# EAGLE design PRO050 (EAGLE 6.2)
CHECKED: PJC; DATE: 9/8/09; DRAWN: PJC; DRGNO: PRO050; REV: A
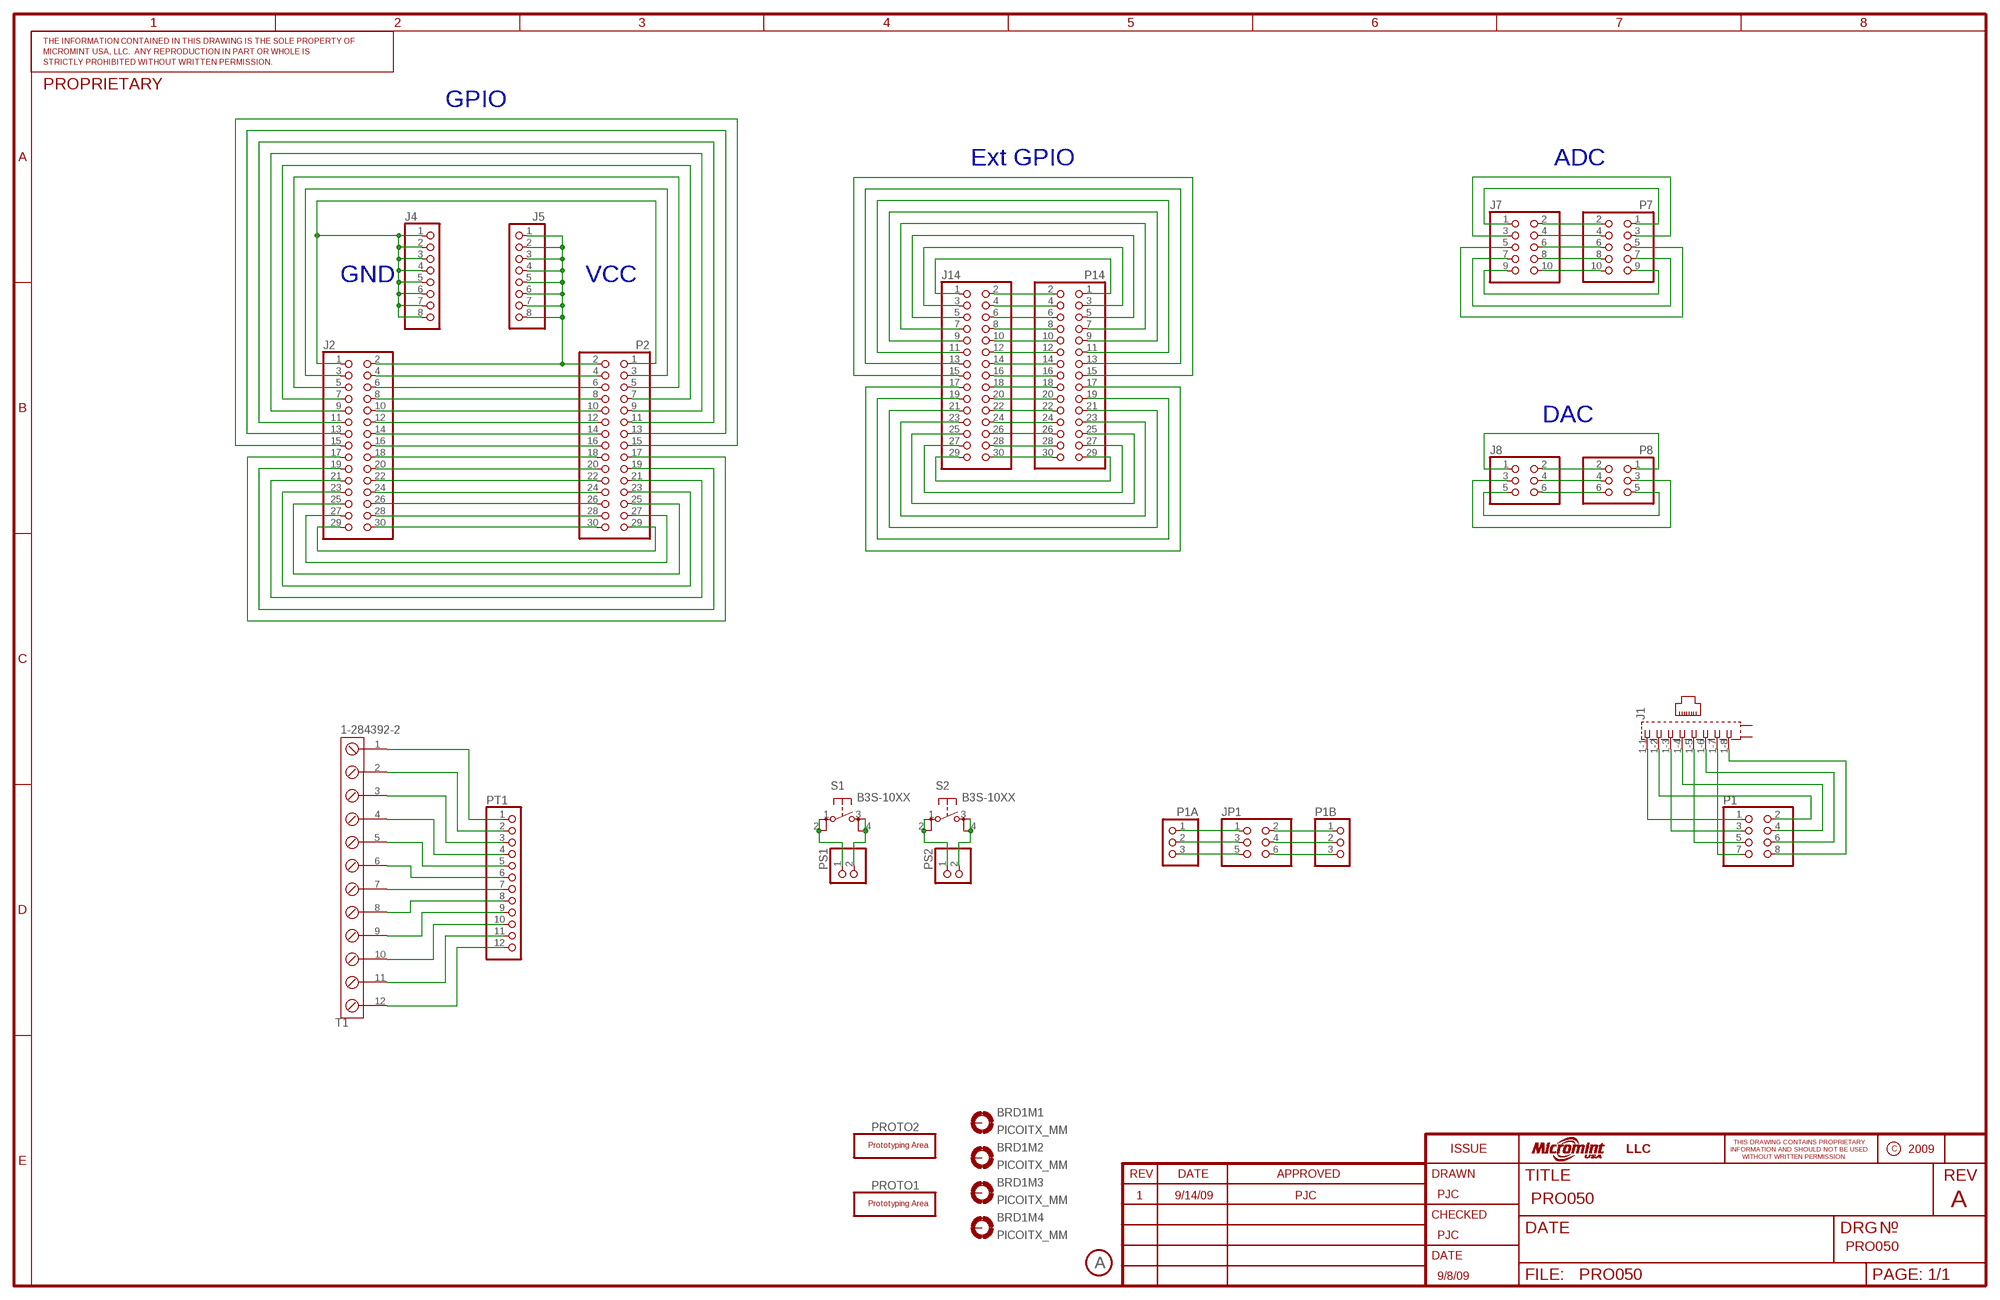
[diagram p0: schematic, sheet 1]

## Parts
BRD1  PICOITX_MM  [PICOITX_MM]
J1  A00-108-262-450  [A00-108-262-450]
J2  PINHD-2X15  [2X15]
J4  PINHD-1X8  [1X08]
J5  PINHD-1X8  [1X08]
J7  PINHD-2X5  [2X05]
J8  PINHD-2X3  [2X03]
J14  PINHD-2X15  [2X15]
JP1  PINHD-2X3  [2X03]
P1  PINHD-2X4  [2X04]
P1A  PINHD-1X3  [1X03]
P1B  PINHD-1X3  [1X03]
P2  PINHD-2X15  [2X15]
P7  PINHD-2X5  [2X05]
P8  PINHD-2X3  [2X03]
P14  PINHD-2X15  [2X15]
PROTO1  PROTO_AREA34X15  [34X15]
PROTO2  PROTO_AREA11X6_MOUNTHOLE  [11X6_MOUNTHOLE]
PS1  PINHD-1X2  [1X02]
PS2  PINHD-1X2  [1X02]
PT1  PINHD-1X12  [1X12]
REV2  A  FIELD_REV-S  [FIELD_REV-S]
S1  B3S-10XX  [B3S-10XX]
S2  B3S-10XX  [B3S-10XX]
T1  1-284392-2  [12POS_0.15_INCHES]

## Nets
N$1: J2.2 J5.1 J5.2 J5.3 J5.4 J5.5 J5.6 J5.7 J5.8 P2.2
N$2: J2.4 P2.4
N$3: J2.6 P2.6
N$4: J2.8 P2.8
N$5: J2.10 P2.10
N$6: J2.12 P2.12
N$7: J2.14 P2.14
N$8: J2.16 P2.16
N$9: J2.18 P2.18
N$10: J2.20 P2.20
N$11: J2.22 P2.22
N$12: J2.24 P2.24
N$13: J2.26 P2.26
N$14: J2.28 P2.28
N$15: J2.30 P2.30
N$16: J14.2 P14.2
N$17: J14.4 P14.4
N$18: J14.6 P14.6
N$19: J14.8 P14.8
N$20: J14.10 P14.10
N$21: J14.12 P14.12
N$22: J14.14 P14.14
N$23: J14.16 P14.16
N$24: J14.18 P14.18
N$25: J14.20 P14.20
N$26: J14.22 P14.22
N$27: J14.24 P14.24
N$28: J14.26 P14.26
N$29: J14.28 P14.28
N$30: J14.30 P14.30
N$31: J14.29 P14.29
N$32: J14.27 P14.27
N$33: J14.25 P14.25
N$34: J14.23 P14.23
N$35: J14.21 P14.21
N$36: J14.19 P14.19
N$37: J14.17 P14.17
N$38: J14.1 P14.1
N$39: PT1.1 T1.1
N$40: J14.3 P14.3
N$41: J14.5 P14.5
N$42: J14.7 P14.7
N$43: J14.9 P14.9
N$44: J14.11 P14.11
N$45: J14.13 P14.13
N$46: J14.15 P14.15
N$47: J2.29 P2.29
N$48: J2.27 P2.27
N$49: J2.25 P2.25
N$50: J2.23 P2.23
N$51: J2.21 P2.21
N$52: J2.19 P2.19
N$53: J2.17 P2.17
N$54: J2.1 J4.1 J4.2 J4.3 J4.4 J4.5 J4.6 J4.7 J4.8 P2.1
N$55: J2.3 P2.3
N$56: J2.5 P2.5
N$57: J2.7 P2.7
N$58: J2.9 P2.9
N$59: J2.11 P2.11
N$60: J2.13 P2.13
N$61: J2.15 P2.15
N$62: PT1.2 T1.2
N$63: PT1.3 T1.3
N$64: PT1.4 T1.4
N$65: PT1.5 T1.5
N$66: PT1.6 T1.6
N$67: PT1.7 T1.7
N$68: PT1.8 T1.8
N$69: PT1.9 T1.9
N$70: PT1.10 T1.10
N$71: PS1.1 S1.1(P) S1.2(P1)
N$72: PS1.2 S1.3(S) S1.4(S1)
N$73: PS2.1 S2.1(P) S2.2(P1)
N$74: PS2.2 S2.3(S) S2.4(S1)
N$75: PT1.11 T1.11
N$76: PT1.12 T1.12
N$77: J1.1-1 P1.1
N$78: J1.1-2 P1.2
N$79: J1.1-3 P1.3
N$80: J1.1-5 P1.5
N$81: J1.1-7 P1.7
N$82: J1.1-4 P1.4
N$83: J1.1-6 P1.6
N$84: J1.1-8 P1.8
N$85: JP1.1 P1A.1
N$86: JP1.3 P1A.2
N$87: JP1.5 P1A.3
N$88: JP1.2 P1B.1
N$89: JP1.4 P1B.2
N$90: JP1.6 P1B.3
N$91: J7.2 P7.2
N$92: J7.4 P7.4
N$93: J7.6 P7.6
N$94: J7.8 P7.8
N$95: J7.10 P7.10
N$96: J7.1 P7.1
N$97: J7.3 P7.3
N$98: J7.9 P7.9
N$99: J7.7 P7.7
N$100: J7.5 P7.5
N$101: J8.2 P8.2
N$102: J8.4 P8.4
N$103: J8.6 P8.6
N$104: J8.1 P8.1
N$105: J8.5 P8.5
N$106: J8.3 P8.3
Unconnected: BRD1.M1 BRD1.M2 BRD1.M3 BRD1.M4 J1.G1(S2) J1.G2(S1)

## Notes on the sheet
- GPIO
- Ext GPIO | ADC
- GND | VCC
- DAC
- 1 | 9/14/09 | PJC
- PRO050

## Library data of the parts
BRD1 = picoitx_mm:PICOITX_MM
J1 = con-edac_MM:A00-108-262-450: EDAC connector
J2 J14 P2 P14 = pinhead:PINHD-2X15: PIN HEADER
J4 J5 = pinhead_MM:PINHD-1X8: PIN HEADER
J7 P7 = pinhead_MM:PINHD-2X5: PIN HEADER
J8 JP1 P8 = pinhead_MM:PINHD-2X3: PIN HEADER
P1 = pinhead_MM:PINHD-2X4: PIN HEADER
P1A P1B = pinhead_MM:PINHD-1X3: PIN HEADER
PROTO1 PROTO2 = proto_MM:PROTO_AREA: Prototyping Areas
PS1 PS2 = pinhead:PINHD-1X2: PIN HEADER
PT1 = pinhead_MM:PINHD-1X12: PIN HEADER
REV2 = micromint_icons:FIELD_REV: Revision Level Field
S1 S2 = switch-omron:B3S-10XX: SMD Tactile Switch
T1 = con-tyco_MM:1-284392-2: Twelve position 0.15" spacing screw terminal

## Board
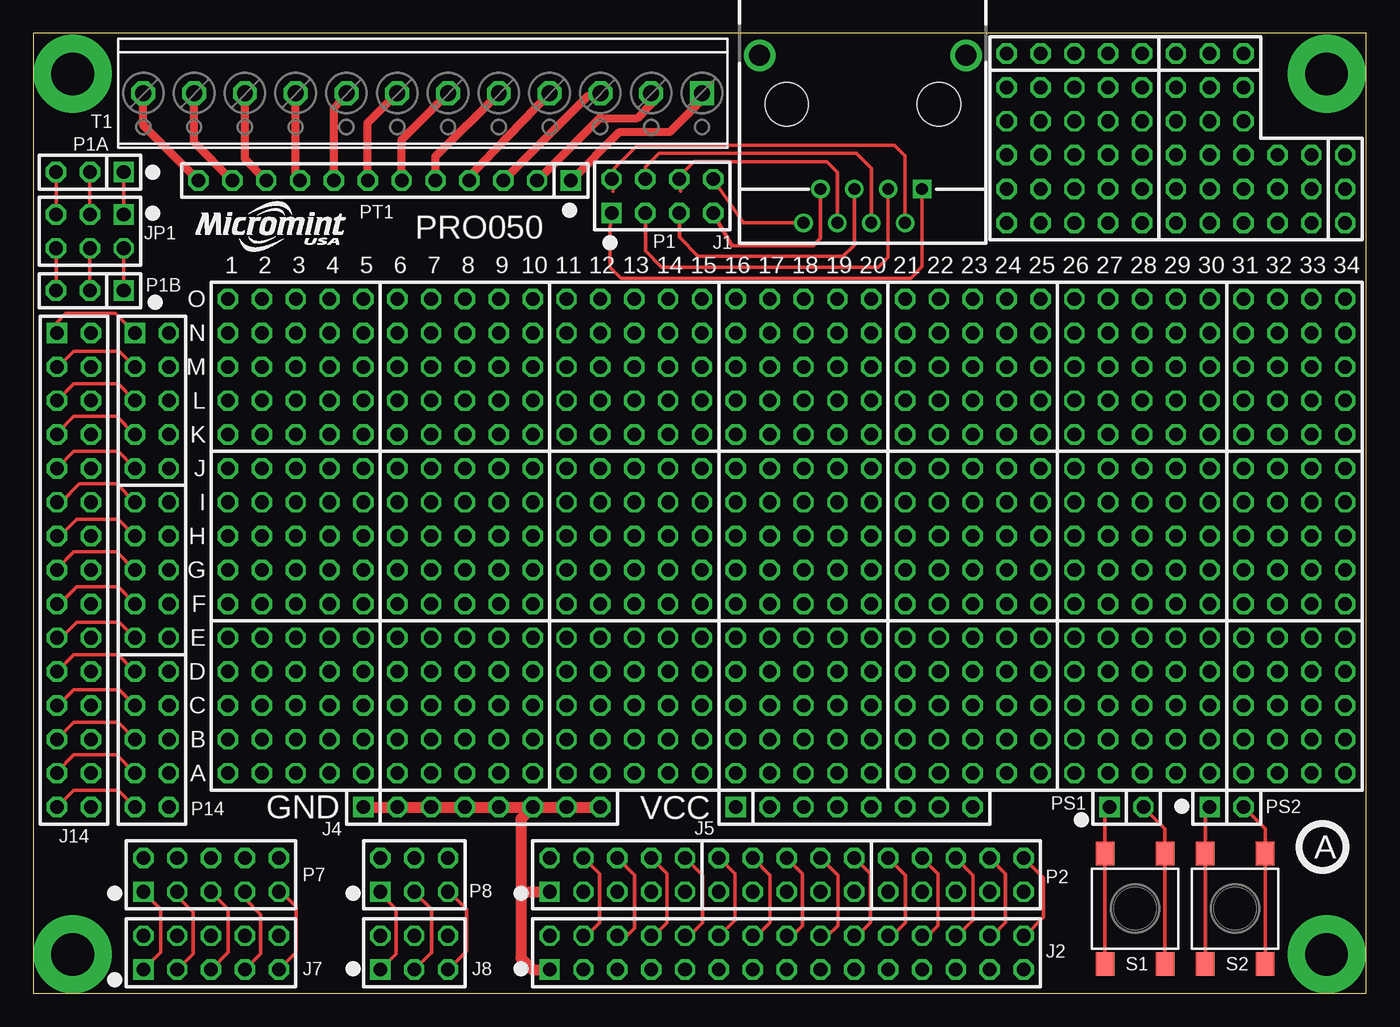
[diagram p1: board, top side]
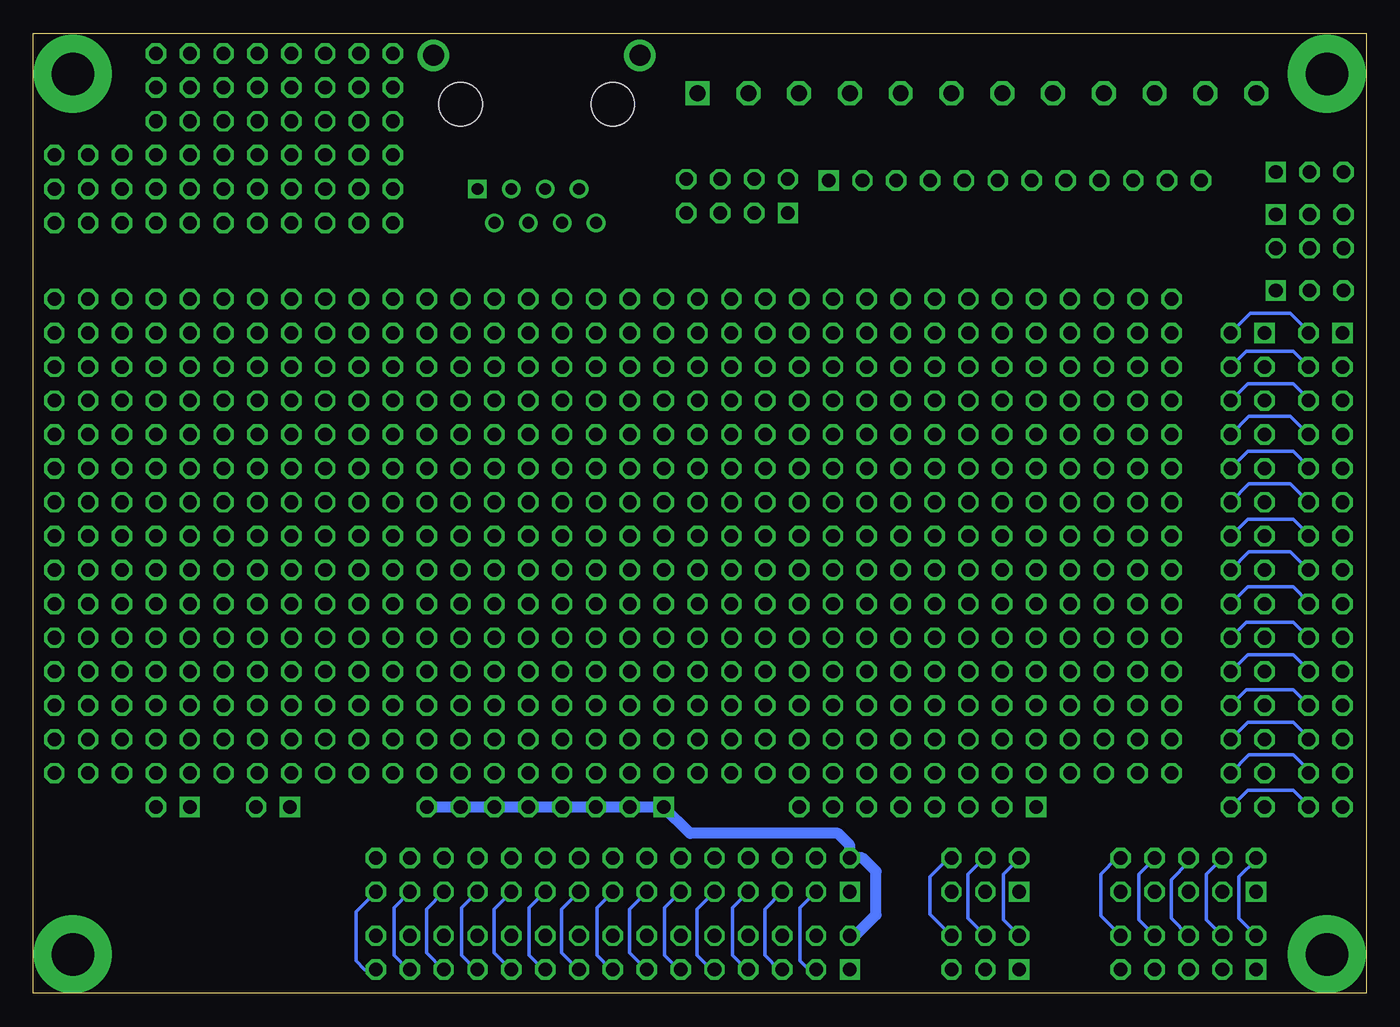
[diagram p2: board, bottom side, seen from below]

Size 100 x 72 mm. Coordinates in mm from the lower left corner, seen from the top.
Copper layers (1*16): Top 0.035mm / dielectric 1.5mm / Bottom 0.035mm
Design rules: minimum track width 10mil, minimum drill 24mil, track to track 10mil, track to pad 10mil, pad to pad 10mil, via to via 10mil, smd to smd 10mil, copper to edge 40mil, drill to drill 8mil, minimum pad ring 10mil, minimum via ring 8mil, stop-mask expansion 4mil, vias tented up to drill 0mil, thermal gap 10mil

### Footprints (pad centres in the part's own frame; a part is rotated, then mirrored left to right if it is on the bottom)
PICOITX_MM = drill 3.2 pad 5.842: M1 2.95,2.92; M2 97.03,2.92; M3 2.95,68.96; M4 97.03,68.96
A00-108-262-450 = drill 0.889 square: 1-1 -4.445,6.35 | drill 0.889: 1-2 -3.175,8.89; 1-3 -1.905,6.35; 1-4 -0.635,8.89; 1-5 0.635,6.35; 1-6 1.905,8.89; 1-7 3.175,6.35; 1-8 4.445,8.89 | drill 1.575 pad 2.184: G1 -7.745,-3.68; G2 7.745,-3.68 | hole 3.251: -5.715,0; 5.715,0
2X15 = drill 1.016 square: 1 -17.78,-1.27 | drill 1.016 octagon: 2 -17.78,1.27; 3 -15.24,-1.27; 4 -15.24,1.27; 5 -12.7,-1.27; 6 -12.7,1.27; 7 -10.16,-1.27; 8 -10.16,1.27; 9 -7.62,-1.27; 10 -7.62,1.27; 11 -5.08,-1.27; 12 -5.08,1.27; 13 -2.54,-1.27; 14 -2.54,1.27; 15 0,-1.27; 16 0,1.27; 17 2.54,-1.27; 18 2.54,1.27; 19 5.08,-1.27; 20 5.08,1.27; 21 7.62,-1.27; 22 7.62,1.27; 23 10.16,-1.27; 24 10.16,1.27; 25 12.7,-1.27; 26 12.7,1.27; 27 15.24,-1.27; 28 15.24,1.27; 29 17.78,-1.27; 30 17.78,1.27
1X08 = drill 1.016 square: 1 -8.89,0 | drill 1.016 octagon: 2 -6.35,0; 3 -3.81,0; 4 -1.27,0; 5 1.27,0; 6 3.81,0; 7 6.35,0; 8 8.89,0
2X05 = drill 1.016 square: 1 -5.08,-1.27 | drill 1.016 octagon: 2 -5.08,1.27; 3 -2.54,-1.27; 4 -2.54,1.27; 5 0,-1.27; 6 0,1.27; 7 2.54,-1.27; 8 2.54,1.27; 9 5.08,-1.27; 10 5.08,1.27
2X03 = drill 1.016 square: 1 -2.54,-1.27 | drill 1.016 octagon: 2 -2.54,1.27; 3 0,-1.27; 4 0,1.27; 5 2.54,-1.27; 6 2.54,1.27
2X04 = drill 1.016 square: 1 -3.81,-1.27 | drill 1.016 octagon: 2 -3.81,1.27; 3 -1.27,-1.27; 4 -1.27,1.27; 5 1.27,-1.27; 6 1.27,1.27; 7 3.81,-1.27; 8 3.81,1.27
1X03 = drill 1.016 square: 1 -2.54,0 | drill 1.016 octagon: 2 0,0; 3 2.54,0
34X15 = drill 1.016 octagon: A1 0,0; A2 2.54,0; A3 5.08,0; A4 7.62,0; A5 10.16,0; A6 12.7,0; A7 15.24,0; A8 17.78,0; A9 20.32,0; A10 22.86,0; A11 25.4,0; A12 27.94,0; A13 30.48,0; A14 33.02,0; A15 35.56,0; A16 38.1,0; A17 40.64,0; A18 43.18,0; A19 45.72,0; A20 48.26,0; A21 50.8,0; A22 53.34,0; A23 55.88,0; A24 58.42,0; A25 60.96,0; A26 63.5,0; A27 66.04,0; A28 68.58,0; A29 71.12,0; A30 73.66,0; A31 76.2,0; A32 78.74,0; A33 81.28,0; A34 83.82,0; B1 0,2.54; B2 2.54,2.54; B3 5.08,2.54; B4 7.62,2.54; B5 10.16,2.54; B6 12.7,2.54; B7 15.24,2.54; B8 17.78,2.54; B9 20.32,2.54; B10 22.86,2.54; B11 25.4,2.54; B12 27.94,2.54; B13 30.48,2.54; B14 33.02,2.54; B15 35.56,2.54; B16 38.1,2.54; B17 40.64,2.54; B18 43.18,2.54; B19 45.72,2.54; B20 48.26,2.54; B21 50.8,2.54; B22 53.34,2.54; B23 55.88,2.54; B24 58.42,2.54; B25 60.96,2.54; B26 63.5,2.54; B27 66.04,2.54; B28 68.58,2.54; B29 71.12,2.54; B30 73.66,2.54; B31 76.2,2.54; B32 78.74,2.54; B33 81.28,2.54; B34 83.82,2.54; C1 0,5.08; C2 2.54,5.08; C3 5.08,5.08; C4 7.62,5.08; C5 10.16,5.08; C6 12.7,5.08; C7 15.24,5.08; C8 17.78,5.08; C9 20.32,5.08; C10 22.86,5.08; C11 25.4,5.08; C12 27.94,5.08; C13 30.48,5.08; C14 33.02,5.08; C15 35.56,5.08; C16 38.1,5.08; C17 40.64,5.08; C18 43.18,5.08; C19 45.72,5.08; C20 48.26,5.08; C21 50.8,5.08; C22 53.34,5.08; C23 55.88,5.08; C24 58.42,5.08; C25 60.96,5.08; C26 63.5,5.08; C27 66.04,5.08; C28 68.58,5.08; C29 71.12,5.08; C30 73.66,5.08; C31 76.2,5.08; C32 78.74,5.08; C33 81.28,5.08; C34 83.82,5.08; D1 0,7.62; D2 2.54,7.62; D3 5.08,7.62; D4 7.62,7.62; D5 10.16,7.62; D6 12.7,7.62; D7 15.24,7.62; D8 17.78,7.62; D9 20.32,7.62; D10 22.86,7.62; D11 25.4,7.62; D12 27.94,7.62; D13 30.48,7.62; D14 33.02,7.62; D15 35.56,7.62; D16 38.1,7.62; D17 40.64,7.62; D18 43.18,7.62; D19 45.72,7.62; D20 48.26,7.62; D21 50.8,7.62; D22 53.34,7.62; D23 55.88,7.62; D24 58.42,7.62; D25 60.96,7.62; D26 63.5,7.62; D27 66.04,7.62; D28 68.58,7.62; D29 71.12,7.62; D30 73.66,7.62; D31 76.2,7.62; D32 78.74,7.62; D33 81.28,7.62; D34 83.82,7.62; E1 0,10.16; E2 2.54,10.16; E3 5.08,10.16; E4 7.62,10.16; E5 10.16,10.16; E6 12.7,10.16; E7 15.24,10.16; E8 17.78,10.16; E9 20.32,10.16; E10 22.86,10.16; E11 25.4,10.16; E12 27.94,10.16; E13 30.48,10.16; E14 33.02,10.16; E15 35.56,10.16; E16 38.1,10.16; E17 40.64,10.16; E18 43.18,10.16; E19 45.72,10.16; E20 48.26,10.16; E21 50.8,10.16; E22 53.34,10.16; E23 55.88,10.16; E24 58.42,10.16; E25 60.96,10.16; E26 63.5,10.16; E27 66.04,10.16; E28 68.58,10.16; E29 71.12,10.16; E30 73.66,10.16; E31 76.2,10.16; E32 78.74,10.16; E33 81.28,10.16; E34 83.82,10.16; F1 0,12.7; F2 2.54,12.7; F3 5.08,12.7; F4 7.62,12.7; F5 10.16,12.7; F6 12.7,12.7; F7 15.24,12.7; F8 17.78,12.7; F9 20.32,12.7; F10 22.86,12.7; F11 25.4,12.7; F12 27.94,12.7; F13 30.48,12.7; F14 33.02,12.7; F15 35.56,12.7; F16 38.1,12.7; F17 40.64,12.7; F18 43.18,12.7; F19 45.72,12.7; F20 48.26,12.7; F21 50.8,12.7; F22 53.34,12.7; F23 55.88,12.7; F24 58.42,12.7; F25 60.96,12.7; F26 63.5,12.7; F27 66.04,12.7; F28 68.58,12.7; F29 71.12,12.7; F30 73.66,12.7; F31 76.2,12.7; F32 78.74,12.7; F33 81.28,12.7; F34 83.82,12.7; G1 0,15.24; G2 2.54,15.24; G3 5.08,15.24; G4 7.62,15.24; G5 10.16,15.24; G6 12.7,15.24; G7 15.24,15.24; G8 17.78,15.24; G9 20.32,15.24; G10 22.86,15.24; G11 25.4,15.24; G12 27.94,15.24; G13 30.48,15.24; G14 33.02,15.24; G15 35.56,15.24; G16 38.1,15.24; G17 40.64,15.24; G18 43.18,15.24; G19 45.72,15.24; G20 48.26,15.24; G21 50.8,15.24; G22 53.34,15.24; G23 55.88,15.24; G24 58.42,15.24; G25 60.96,15.24; G26 63.5,15.24; G27 66.04,15.24; G28 68.58,15.24; G29 71.12,15.24; G30 73.66,15.24; G31 76.2,15.24; G32 78.74,15.24; G33 81.28,15.24; G34 83.82,15.24; H1 0,17.78; H2 2.54,17.78; H3 5.08,17.78; H4 7.62,17.78; H5 10.16,17.78; H6 12.7,17.78; H7 15.24,17.78; H8 17.78,17.78; H9 20.32,17.78; H10 22.86,17.78; H11 25.4,17.78; H12 27.94,17.78; H13 30.48,17.78; H14 33.02,17.78; H15 35.56,17.78; H16 38.1,17.78; H17 40.64,17.78; H18 43.18,17.78; H19 45.72,17.78; H20 48.26,17.78; H21 50.8,17.78; H22 53.34,17.78; H23 55.88,17.78; H24 58.42,17.78; H25 60.96,17.78; H26 63.5,17.78; H27 66.04,17.78; H28 68.58,17.78; H29 71.12,17.78; H30 73.66,17.78; H31 76.2,17.78; H32 78.74,17.78; H33 81.28,17.78; H34 83.82,17.78; I1 0,20.32; I2 2.54,20.32; I3 5.08,20.32; I4 7.62,20.32; I5 10.16,20.32; I6 12.7,20.32; I7 15.24,20.32; I8 17.78,20.32; I9 20.32,20.32; I10 22.86,20.32; I11 25.4,20.32; I12 27.94,20.32; I13 30.48,20.32; I14 33.02,20.32; I15 35.56,20.32; I16 38.1,20.32; I17 40.64,20.32; I18 43.18,20.32; I19 45.72,20.32; I20 48.26,20.32; I21 50.8,20.32; I22 53.34,20.32; I23 55.88,20.32; I24 58.42,20.32; I25 60.96,20.32; I26 63.5,20.32; I27 66.04,20.32; I28 68.58,20.32; I29 71.12,20.32; I30 73.66,20.32; I31 76.2,20.32; I32 78.74,20.32; I33 81.28,20.32; I34 83.82,20.32; J1 0,22.86; J2 2.54,22.86; J3 5.08,22.86; J4 7.62,22.86; J5 10.16,22.86; J6 12.7,22.86; J7 15.24,22.86; J8 17.78,22.86; J9 20.32,22.86; J10 22.86,22.86; J11 25.4,22.86; J12 27.94,22.86; J13 30.48,22.86; J14 33.02,22.86; J15 35.56,22.86; J16 38.1,22.86; J17 40.64,22.86; J18 43.18,22.86; J19 45.72,22.86; J20 48.26,22.86; J21 50.8,22.86; J22 53.34,22.86; J23 55.88,22.86; J24 58.42,22.86; J25 60.96,22.86; J26 63.5,22.86; J27 66.04,22.86; J28 68.58,22.86; J29 71.12,22.86; J30 73.66,22.86; J31 76.2,22.86; J32 78.74,22.86; J33 81.28,22.86; J34 83.82,22.86; K1 0,25.4; K2 2.54,25.4; K3 5.08,25.4; K4 7.62,25.4; K5 10.16,25.4; K6 12.7,25.4; K7 15.24,25.4; K8 17.78,25.4; K9 20.32,25.4; K10 22.86,25.4; K11 25.4,25.4; K12 27.94,25.4; K13 30.48,25.4; K14 33.02,25.4; K15 35.56,25.4; K16 38.1,25.4; K17 40.64,25.4; K18 43.18,25.4; K19 45.72,25.4; K20 48.26,25.4; K21 50.8,25.4; K22 53.34,25.4; K23 55.88,25.4; K24 58.42,25.4; K25 60.96,25.4; K26 63.5,25.4; K27 66.04,25.4; K28 68.58,25.4; K29 71.12,25.4; K30 73.66,25.4; K31 76.2,25.4; K32 78.74,25.4; K33 81.28,25.4; K34 83.82,25.4; L1 0,27.94; L2 2.54,27.94; L3 5.08,27.94; L4 7.62,27.94; L5 10.16,27.94; L6 12.7,27.94; L7 15.24,27.94; L8 17.78,27.94; L9 20.32,27.94; L10 22.86,27.94; L11 25.4,27.94; L12 27.94,27.94; L13 30.48,27.94; L14 33.02,27.94; L15 35.56,27.94; L16 38.1,27.94; L17 40.64,27.94; L18 43.18,27.94; L19 45.72,27.94; L20 48.26,27.94; L21 50.8,27.94; L22 53.34,27.94; L23 55.88,27.94; L24 58.42,27.94; L25 60.96,27.94; L26 63.5,27.94; L27 66.04,27.94; L28 68.58,27.94; L29 71.12,27.94; L30 73.66,27.94; L31 76.2,27.94; L32 78.74,27.94; L33 81.28,27.94; L34 83.82,27.94; M1 0,30.48; M2 2.54,30.48; M3 5.08,30.48; M4 7.62,30.48; M5 10.16,30.48; M6 12.7,30.48; M7 15.24,30.48; M8 17.78,30.48; M9 20.32,30.48; M10 22.86,30.48; M11 25.4,30.48; M12 27.94,30.48; M13 30.48,30.48; M14 33.02,30.48; M15 35.56,30.48; M16 38.1,30.48; M17 40.64,30.48; M18 43.18,30.48; M19 45.72,30.48; M20 48.26,30.48; M21 50.8,30.48; M22 53.34,30.48; M23 55.88,30.48; M24 58.42,30.48; M25 60.96,30.48; M26 63.5,30.48; M27 66.04,30.48; M28 68.58,30.48; M29 71.12,30.48; M30 73.66,30.48; M31 76.2,30.48; M32 78.74,30.48; M33 81.28,30.48; M34 83.82,30.48; N1 0,33.02; N2 2.54,33.02; N3 5.08,33.02; N4 7.62,33.02; N5 10.16,33.02; N6 12.7,33.02; N7 15.24,33.02; N8 17.78,33.02; N9 20.32,33.02; N10 22.86,33.02; N11 25.4,33.02; N12 27.94,33.02; N13 30.48,33.02; N14 33.02,33.02; N15 35.56,33.02; N16 38.1,33.02; N17 40.64,33.02; N18 43.18,33.02; N19 45.72,33.02; N20 48.26,33.02; N21 50.8,33.02; N22 53.34,33.02; N23 55.88,33.02; N24 58.42,33.02; N25 60.96,33.02; N26 63.5,33.02; N27 66.04,33.02; N28 68.58,33.02; N29 71.12,33.02; N30 73.66,33.02; N31 76.2,33.02; N32 78.74,33.02; N33 81.28,33.02; N34 83.82,33.02; O1 0,35.56; O2 2.54,35.56; O3 5.08,35.56; O4 7.62,35.56; O5 10.16,35.56; O6 12.7,35.56; O7 15.24,35.56; O8 17.78,35.56; O9 20.32,35.56; O10 22.86,35.56; O11 25.4,35.56; O12 27.94,35.56; O13 30.48,35.56; O14 33.02,35.56; O15 35.56,35.56; O16 38.1,35.56; O17 40.64,35.56; O18 43.18,35.56; O19 45.72,35.56; O20 48.26,35.56; O21 50.8,35.56; O22 53.34,35.56; O23 55.88,35.56; O24 58.42,35.56; O25 60.96,35.56; O26 63.5,35.56; O27 66.04,35.56; O28 68.58,35.56; O29 71.12,35.56; O30 73.66,35.56; O31 76.2,35.56; O32 78.74,35.56; O33 81.28,35.56; O34 83.82,35.56
11X6_MOUNTHOLE = drill 1.016 octagon: A1 0,0; A2 2.54,0; A3 5.08,0; A4 7.62,0; A5 10.16,0; A6 12.7,0; A7 15.24,0; A8 17.78,0; A9 20.32,0; A10 22.86,0; A11 25.4,0; B1 0,2.54; B2 2.54,2.54; B3 5.08,2.54; B4 7.62,2.54; B5 10.16,2.54; B6 12.7,2.54; B7 15.24,2.54; B8 17.78,2.54; B9 20.32,2.54; B10 22.86,2.54; B11 25.4,2.54; C1 0,5.08; C2 2.54,5.08; C3 5.08,5.08; C4 7.62,5.08; C5 10.16,5.08; C6 12.7,5.08; C7 15.24,5.08; C8 17.78,5.08; C9 20.32,5.08; C10 22.86,5.08; C11 25.4,5.08; D1 0,7.62; D2 2.54,7.62; D3 5.08,7.62; D4 7.62,7.62; D5 10.16,7.62; D6 12.7,7.62; D7 15.24,7.62; D8 17.78,7.62; E1 0,10.16; E2 2.54,10.16; E3 5.08,10.16; E4 7.62,10.16; E5 10.16,10.16; E6 12.7,10.16; E7 15.24,10.16; E8 17.78,10.16; F1 0,12.7; F2 2.54,12.7; F3 5.08,12.7; F4 7.62,12.7; F5 10.16,12.7; F6 12.7,12.7; F7 15.24,12.7; F8 17.78,12.7
1X02 = drill 1.016 square: 1 -1.27,0 | drill 1.016 octagon: 2 1.27,0
1X12 = drill 1.016 square: 1 -13.97,0 | drill 1.016 octagon: 2 -11.43,0; 3 -8.89,0; 4 -6.35,0; 5 -3.81,0; 6 -1.27,0; 7 1.27,0; 8 3.81,0; 9 6.35,0; 10 8.89,0; 11 11.43,0; 12 13.97,0
B3S-10XX = smd 1.75 x 1.4: 1 -4.15,2.25; 2 4.15,2.25; 3 -4.15,-2.25; 4 4.15,-2.25
12POS_0.15_INCHES = drill 1.194 square: 1 -20.955,0 | drill 1.194 octagon: 2 -17.145,0; 3 -13.335,0; 4 -9.525,0; 5 -5.715,0; 6 -1.905,0; 7 1.905,0; 8 5.715,0; 9 9.525,0; 10 13.335,0; 11 17.145,0; 12 20.955,0

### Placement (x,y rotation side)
BRD1  0,0 0 top
J1  62.23,66.67 180 top
J2  56.52,3.05 0 top
J4  33.66,13.97 0 top
J5  61.59,13.97 0 top
J7  13.34,3.05 0 top
J8  28.57,3.05 0 top
J14  3.05,31.75 270 top
JP1  4.24,57.15 180 top
P1  47.19,59.79 0 top
P1A  4.24,61.59 180 top
P1B  4.24,52.7 180 top
P2  56.52,8.89 0 top
P7  13.34,8.89 0 top
P8  28.57,8.89 0 top
P14  8.89,31.75 270 top
PROTO1  14.61,16.51 0 top
PROTO2  73.03,57.78 0 top
PS1  82.02,13.97 0 top
PS2  89.53,13.97 0 top
PT1  26.37,60.96 180 top
REV2  96.72,10.97 0 top
S1  82.65,6.35 90 top
S2  90.17,6.35 90 top
T1  29.21,67.51 180 top
U$1  [LOGO_M]  17.63,57.56 0 top
U$2  [PIN1]  23.98,1.83 0 top
U$3  [PIN1]  23.98,7.52 0 top
U$4  [PIN1]  36.58,7.52 0 top
U$5  [PIN1]  36.58,1.83 0 top
U$6  [PIN1]  6.1,1.02 0 top
U$7  [PIN1]  6.1,7.52 0 top
U$8  [PIN1]  9.14,51.82 0 top
U$9  [PIN1]  86.16,14.02 0 top
U$10  [PIN1]  78.64,13 0 top
U$11  [PIN1]  43.28,56.29 0 top
U$12  [PIN1]  40.23,58.72 0 top
U$13  [PIN1]  8.94,58.52 0 top
U$14  [PIN1]  8.94,61.57 0 top

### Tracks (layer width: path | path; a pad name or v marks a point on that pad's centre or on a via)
N$1
  Bottom 0.813: J2.2 38.35,4.32 36.78,5.89 36.78,9.14 37.8,10.16 P2.2 38.73,11.1 39.62,11.99 50.72,11.99 J5.1 J5.2 55.3,14.02 55.68,14.02 55.73,13.97 J5.3 J5.4 J5.5 J5.6 J5.7 J5.8
N$2
  Top 0.254: J2.4 41.5,4.32 42.47,5.28 42.47,8.97 P2.4
N$3
  Top 0.254: J2.6 44.55,4.32 45.11,4.88 45.11,8.87 P2.6
N$4
  Top 0.254: J2.8 46.58,4.32 47.55,5.28 47.55,8.97 P2.8
N$5
  Top 0.254: J2.10 49.23,4.32 50.19,5.28 50.19,8.87 P2.10
N$6
  Top 0.254: J2.12 51.46,4.32 52.63,5.49 52.63,8.97 P2.12
N$7
  Top 0.254: J2.14 54.3,4.32 55.27,5.28 55.27,8.87 P2.14
N$8
  Top 0.254: J2.16 56.95,4.32 57.71,5.08 57.71,8.97 P2.16
N$9
  Top 0.254: J2.18 59.59,4.32 60.35,5.08 60.35,8.87 P2.18
N$10
  Top 0.254: J2.20 61.82,4.32 62.79,5.28 62.79,8.97 P2.20
N$11
  Top 0.254: J2.22 64.47,4.32 65.43,5.28 65.43,8.87 P2.22
N$12
  Top 0.254: J2.24 67.11,4.32 67.87,5.08 67.87,8.97 P2.24
N$13
  Top 0.254: J2.26 69.34,4.32 70.51,5.49 70.51,8.87 P2.26
N$14
  Top 0.254: J2.28 71.98,4.32 72.95,5.28 72.95,8.97 P2.28
N$15
  Top 0.254: J2.30 74.42,4.32 75.79,5.69 75.79,8.66 P2.30
N$16
  Bottom 0.254: J14.2 4.32,49.63 5.69,51 8.69,51 P14.2
N$17
  Bottom 0.254: J14.4 5.49,48.16 8.99,48.16 P14.4
N$18
  Bottom 0.254: J14.6 4.32,44.55 5.49,45.72 8.89,45.72 P14.6
N$19
  Bottom 0.254: J14.8 5.69,43.28 8.79,43.28 P14.8
N$20
  Bottom 0.254: J14.10 4.32,39.47 5.49,40.64 8.89,40.64 P14.10
N$21
  Bottom 0.254: J14.12 5.69,38.2 8.79,38.2 P14.12
N$22
  Bottom 0.254: J14.14 4.32,34.39 5.49,35.56 8.89,35.56 P14.14
N$23
  Bottom 0.254: J14.16 5.69,33.12 8.79,33.12 P14.16
N$24
  Bottom 0.254: J14.18 4.32,29.31 5.49,30.48 8.89,30.48 P14.18
N$25
  Bottom 0.254: J14.20 5.49,27.84 8.99,27.84 P14.20
N$26
  Bottom 0.254: J14.22 4.32,24.23 5.49,25.4 8.89,25.4 P14.22
N$27
  Bottom 0.254: J14.24 5.49,22.76 8.99,22.76 P14.24
N$28
  Bottom 0.254: J14.26 4.32,19.15 5.49,20.32 8.89,20.32 P14.26
N$29
  Bottom 0.254: J14.28 4.32,16.71 5.49,17.88 8.79,17.88 P14.28
N$30
  Bottom 0.254: J14.30 4.32,14.07 5.49,15.24 8.89,15.24 P14.30
N$31
  Top 0.254: J14.29 3.05,15.24 6.35,15.24 P14.29
N$32
  Top 0.254: J14.27 1.78,16.61 3.05,17.88 6.25,17.88 P14.27
N$33
  Top 0.254: J14.25 3.05,20.32 6.35,20.32 P14.25
N$34
  Top 0.254: J14.23 1.88,21.59 3.05,22.76 6.45,22.76 P14.23
N$35
  Top 0.254: J14.21 3.05,25.4 6.35,25.4 P14.21
N$36
  Top 0.254: J14.19 2.08,26.67 3.25,27.84 6.45,27.84 P14.19
N$37
  Top 0.254: J14.17 1.98,29.21 3.25,30.48 6.35,30.48 P14.17
N$38
  Top 0.254: J14.1 1.78,50.34 2.44,51 6.15,51 P14.1
N$39
  Top 0.61: PT1.1 43.99,64.62 47.75,64.62 50.16,67.03 T1.1
N$40
  Top 0.254: J14.3 1.88,46.99 3.05,48.16 6.45,48.16 P14.3
N$41
  Top 0.254: J14.5 3.05,45.72 6.35,45.72 P14.5
N$42
  Top 0.254: J14.7 1.78,42.01 3.05,43.28 6.25,43.28 P14.7
N$43
  Top 0.254: J14.9 3.05,40.64 6.35,40.64 P14.9
N$44
  Top 0.254: J14.11 2.08,36.83 3.45,38.2 6.25,38.2 P14.11
N$45
  Top 0.254: J14.13 1.98,34.29 3.25,35.56 6.35,35.56 P14.13
N$46
  Top 0.254: J14.15 1.78,31.85 3.05,33.12 6.25,33.12 P14.15
N$47
  Bottom 0.254: J2.29 75.13,1.78 75.79,2.44 75.79,6.12 P2.29
N$48
  Bottom 0.254: J2.27 71.88,1.78 72.95,2.85 72.95,6.43 P2.27
N$49
  Bottom 0.254: J2.25 69.24,1.78 70.51,3.05 70.51,6.33 P2.25
N$50
  Bottom 0.254: J2.23 66.8,1.78 67.87,2.85 67.87,6.43 P2.23
N$51
  Bottom 0.254: J2.21 64.16,1.78 65.43,3.05 65.43,6.33 P2.21
N$52
  Bottom 0.254: J2.19 61.72,1.78 62.79,2.85 62.79,6.43 P2.19
N$53
  Bottom 0.254: J2.17 59.08,1.78 60.35,3.05 60.35,6.33 P2.17
N$54
  Top 0.813: J2.1 37.44,1.78 36.58,2.64 36.58,7.52 | 36.58,7.52 36.58,13.08 J4.6 | J4.8 J4.7 J4.6 | J4.1 J4.2 J4.3 J4.4 J4.5 J4.6 | P2.1 36.68,7.62 36.58,7.52
N$55
  Bottom 0.254: J2.3 41.81,1.78 42.47,2.44 42.47,6.43 P2.3
N$56
  Bottom 0.254: J2.5 44.04,1.78 45.11,2.85 45.11,6.33 P2.5
N$57
  Bottom 0.254: J2.7 46.48,1.78 47.55,2.85 47.55,6.43 P2.7
N$58
  Bottom 0.254: J2.9 49.12,1.78 50.19,2.85 50.19,6.33 P2.9
N$59
  Bottom 0.254: J2.11 51.56,1.78 52.63,2.85 52.63,6.43 P2.11
N$60
  Bottom 0.254: J2.13 54,1.78 55.27,3.05 55.27,6.33 P2.13
N$61
  Bottom 0.254: J2.15 56.64,1.78 57.71,2.85 57.71,6.43 P2.15
N$62
  Top 0.61: PT1.2 42.47,65.63 45.31,65.63 46.35,66.67 T1.2
N$63
  Top 0.61: PT1.3 41.6,67.31 T1.3
N$64
  Top 0.61: PT1.4 32.72,61.29 T1.4
N$65
  Top 0.61: PT1.5 30.18,62.76 T1.5
N$66
  Top 0.61: PT1.6 27.64,64.03 T1.6
N$67
  Top 0.61: PT1.7 25.09,65.3 T1.7
N$68
  Top 0.61: PT1.8 22.55,66.37 T1.8
N$69
  Top 0.61: PT1.9 19.68,61.29 T1.9
N$70
  Top 0.61: PT1.10 15.88,62.56 T1.10
N$71
  Top 0.254: S1.1 S1.2 80.4,13.62 PS1.1
N$72
  Top 0.254: S1.3 S1.4 84.9,12.36 PS1.2
N$73
  Top 0.254: S2.1 S2.2 87.92,13.62 PS2.1
N$74
  Top 0.254: S2.3 S2.4 92.42,12.36 PS2.2
N$75
  Top 0.61: PT1.11 12.06,63.83 T1.11
N$76
  Top 0.61: PT1.12 8.26,65.1 T1.12
N$77
  Top 0.254: J1.1-1 66.67,54.48 65.84,53.65 44.09,53.65 43.28,54.46 43.28,57.4 P1.1
N$78
  Top 0.254: J1.1-2 65.41,62.81 64.62,63.6 45.31,63.6 43.48,61.77 43.48,60.15 P1.2
N$79
  Top 0.254: J1.1-3 64.14,55.19 63.4,54.46 47.14,54.46 45.92,55.68 P1.3
N$80
  Top 0.254: J1.1-5 61.59,56.11 60.76,55.27 49.89,55.27 48.46,56.69 P1.5
N$81
  Top 0.254: J1.1-7 59.05,56.62 58.52,56.08 52.43,56.08 P1.7
N$82
  Top 0.254: J1.1-4 62.87,61.9 61.77,62.99 46.94,62.99 45.92,61.98 P1.4
N$83
  Top 0.254: J1.1-6 60.33,61.59 59.54,62.38 49.58,62.38 48.56,61.37 48.56,60.15 P1.6
N$84
  Top 0.254: J1.1-8 53.26,57.78 P1.8
N$85
  Top 0.254: JP1.1 P1A.1
N$86
  Top 0.254: JP1.3 P1A.2
N$87
  Top 0.254: JP1.5 P1A.3
N$88
  Top 0.254: P1B.1 JP1.2
N$89
  Top 0.254: P1B.2 JP1.4
N$90
  Top 0.254: P1B.3 JP1.6
N$91
  Bottom 0.254: J7.2 9.55,5.61 9.55,8.74 8.26,10.03 P7.2
N$92
  Bottom 0.254: J7.4 11.99,5.51 11.99,8.94 10.79,10.13 P7.4
N$93
  Bottom 0.254: J7.6 14.63,5.61 14.63,8.53 13.34,9.83 P7.6
N$94
  Bottom 0.254: J7.8 17.07,5.51 17.07,8.94 15.88,10.13 P7.8
N$95
  Bottom 0.254: J7.10 19.91,5.82 19.91,8.94 18.69,10.16 P7.10
N$96
  Top 0.254: J7.1 9.55,3.07 9.55,6.3 8.26,7.59 P7.1
N$97
  Top 0.254: J7.3 11.99,2.97 11.99,6.1 10.79,7.29 P7.3
N$98
  Top 0.254: J7.9 19.71,3.07 19.71,6.5 18.59,7.62 P7.9
N$99
  Top 0.254: J7.7 17.07,2.97 17.07,5.89 15.88,7.09 P7.7
N$100
  Top 0.254: J7.5 14.63,3.07 14.63,6.3 13.34,7.59 P7.5
N$101
  Bottom 0.254: J8.2 27.23,5.51 27.23,8.94 26.04,10.13 P8.2
N$102
  Bottom 0.254: J8.4 29.87,5.61 29.87,8.94 28.65,10.16 P8.4
N$103
  Bottom 0.254: J8.6 32.72,5.92 32.72,8.74 31.29,10.16 P8.6
N$104
  Top 0.254: J8.1 27.23,2.97 27.23,6.3 26.04,7.49 P8.1
N$105
  Top 0.254: J8.5 32.51,3.17 32.51,6.3 31.19,7.62 P8.5
N$106
  Top 0.254: J8.3 29.84,3.05 29.87,3.05 29.87,6.3 28.57,7.59 P8.3

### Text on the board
tPlace: PRO050 | GND | VCC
